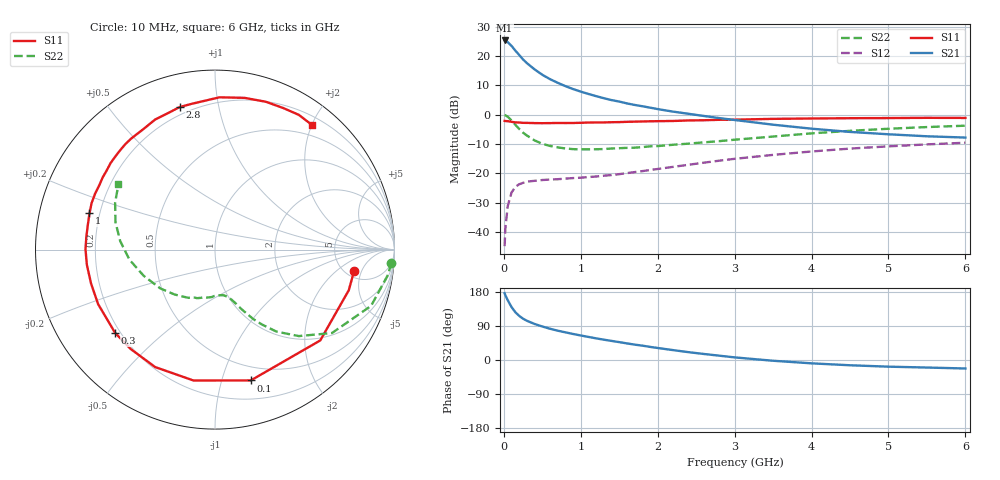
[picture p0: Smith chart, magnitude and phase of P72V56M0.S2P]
! SIEMENS Small Signal Semiconductors
! BFP196
! Si NPN RF Bipolar Junction Transistor in SOT143
! VCE = 2.5 V  IC = 6 mA
! Common Emitter S-Parameters:  May  1996
# GHz  S  MA  R  50
!  f  S11  S21  S12  S22
! GHz  MAG  ANG  MAG  ANG  MAG  ANG  MAG  ANG
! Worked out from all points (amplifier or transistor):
!   36 points, 10 MHz to 6 GHz, reference 50 ohm
!   highest |S21| = 25.3 dB at 10 MHz (marker M1)
!   |S21| within 3 dB of that: start of sweep to 135.4 MHz
!   unconditionally stable (mu >= 1): 1.054 GHz to 3.282 GHz; 5.951 GHz to end of sweep
!   at 250 MHz: K = 0.29, MSG = 21.1 dB, |S12| = -23.3 dB
!   at 1.4 GHz: K = 1.17, MAG = 10.3 dB, |S12| = -20.6 dB
!   at 6 GHz: K = 1.00, MAG = 0.6 dB, |S12| = -9.6 dB
!   S11 on the Smith chart (normalised r, x): 10 MHz: 5.96, -3.67; 100 MHz: 0.37, -1.24; 300 MHz: 0.18, -0.35; 1 GHz: 0.16, +0.14; 2.8 GHz: 0.16, +0.77; 6 GHz: 0.32, +1.99
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0.01  0.7841 -8.7  18.5 176.4  0.0057 86.9  0.9846 -4.3
0.02  0.779 -16.9  18.12 170.6  0.0116 79.2  0.9746 -8.2
0.05  0.7746 -40.8  17.35 157.9  0.0273 69.5  0.9245 -19.8
0.1  0.7557 -74.7  14.95 139.8  0.047 54.8  0.8005 -35.5
0.15  0.7391 -99.3  12.39 125.9  0.0586 44.2  0.671 -45.9
0.2  0.7345 -117.0  10.44 116.4  0.065 37.2  0.5702 -53.2
0.25  0.7262 -130.4  8.762 109.0  0.0687 32.5  0.4929 -57.9
0.3  0.7245 -140.2  7.581 103.5  0.072 29.9  0.4409 -61.2
0.4  0.7186 -155.0  5.929 95.1  0.0744 26.4  0.3636 -66.0
0.5  0.716 -164.8  4.799 88.4  0.0767 24.9  0.3187 -69.2
0.6  0.7189 -173.2  4.045 82.5  0.0782 24.4  0.2931 -71.8
0.8  0.7204 174.3  3.073 73.0  0.0811 25.5  0.2652 -77.0
1  0.7278 163.9  2.475 64.7  0.0841 27.8  0.2562 -82.3
1.1  0.7346 159.4  2.259 60.9  0.0862 29.1  0.2564 -85.3
1.3  0.7376 150.9  1.911 53.6  0.0909 31.8  0.2589 -91.1
1.6  0.7557 140.3  1.558 43.8  0.1007 35.6  0.2714 -100.4
2.2  0.7809 120.8  1.128 26.1  0.1287 39.9  0.3069 -118.9
2.8  0.8182 103.9  0.876 11.4  0.164 38.6  0.3535 -138.8
3.5  0.8489 88.3  0.675 -2.0  0.2061 32.8  0.4235 -159.9
4.5  0.871 71.0  0.508 -13.9  0.2639 21.7  0.5301 174.9
5.5  0.8841 58.1  0.428 -19.9  0.3113 9.6  0.615 154.8
6  0.8799 52.3  0.407 -22.4  0.3321 3.0  0.649 146.0
